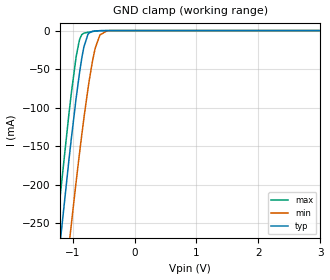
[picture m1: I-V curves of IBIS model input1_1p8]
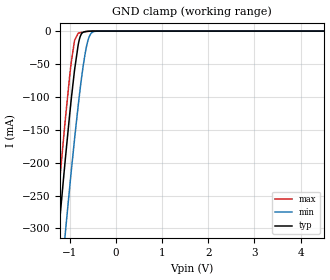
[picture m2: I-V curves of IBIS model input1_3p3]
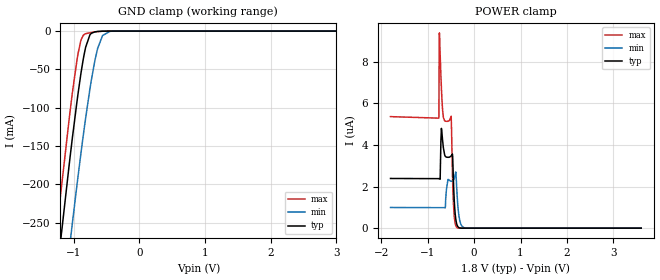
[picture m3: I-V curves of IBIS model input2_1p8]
| Texas Instruments Incorporated
| TLV320ADC5140 Quad-Channel, 768-kHz, Burr-Brown Audio ADC
[IBIS Ver]   4.1
[File name]   tlv320adc5140.ibs
[Date]   05/10/2019
[File Rev]   1.0
[Source]
| Texas Instruments Incorporated.
| Analog-eLab Design Center, HPA
| 12500 TI Blvd
| Dallas, TX -75243
[Notes]   Revision History:
| Rev 1.0: 05/10/2019
| - Initial version of the model
| - Model generated from simulations in SPECTRE
| - C_comp although listed in numerical order of value are
|   obtained from varying PVT conditions. For PVT conditions for
|   each specific value refer the buffer description under
|   respective [Model]. IBIS model user is responsible for using
|   appropriate C_comp to simulate for Signal Integrity.
| - Warnings regarding combined Non-monotonicity of various models have been
|   reviewd and considered minor and can be ignored.
| - Model names with a trailing _1p8 contain the model for 1.8V operation.
|   Model names with a trailing _3p3 contain the model for 3.3V operation.
[Disclaimer]
| This model is designed as an aid for customers of Texas Instruments.
| TI and its licensors and suppliers make no warranties, either expressed
| or implied, with respect to this  model, including the warranties of
| merchantability or fitness for a particular purpose. The model is
| provided solely on an "as is" basis. The entire risk as to its quality
| and performance is with the customer.
| This model is subject to change without notice. Texas Instruments
| Incorporated is not responsible for updating this model.
[Copyright]
(C) Copyright 2019 Texas Instruments Incorporated.All rights reserved.
|  Component TLV320ADC5140RTW 24-Pin WQFN - RTW package
|  Part # TLV320ADC5140RTW
[Component]   TLV320ADC5140RTW
[Manufacturer]  TI
[Package]   |24 WQFN - RTW package
|   typ   min   max
R_pkg   0.05   0.04   0.06
L_pkg   1.0nH   0.8nH   1.2nH
C_pkg   0.2pF   0.16pF   0.24pF
[Pin]  signal_name   model_name   R_pin   L_pin   C_pin
1   AVDD   power   NA   NA   NA
2   AREG   power   NA   NA   NA
3   VREF   nc   NA   NA   NA
4   AVSS   gnd   NA   NA   NA
5   MICBIAS   nc   NA   NA   NA
6   IN1P_GPI1   input1   NA   NA   NA
7   IN1M_GPO1   output   NA   NA   NA
8   IN2P_GPI2   input1   NA   NA   NA
9   IN2M_GPO2   output   NA   NA   NA
10   IN3P_GPI3   input1   NA   NA   NA
11   IN3M_GPO3   output   NA   NA   NA
12   IN4P_GPI4   input1   NA   NA   NA
13   IN4M_GPO4   output   NA   NA   NA
14   SHDNZ   input3   NA   NA   NA
15   ADDR1_MISO   io   NA   NA   NA
16   ADDR0_SCLK   input2   NA   NA   NA
17   SCL_MOSI   od   NA   NA   NA
18   SDA_SSZ   od   NA   NA   NA
19   IOVDD   power   NA   NA   NA
20   GPIO1   io   NA   NA   NA
21   SDOUT   io   NA   NA   NA
22   BCLK   io   NA   NA   NA
23   FSYNC   io   NA   NA   NA
24   DREG   power   NA   NA   NA
|   Model Selectors
[Model Selector] input1
input1_1p8   1.8V   digital Input
input1_3p3   3.3V   digital Input
[Model Selector] input2
input2_1p8   1.8V   digital Input
input2_3p3   3.3V   digital Input
[Model Selector] input3
input3_1p8   1.8V   digital Input
input3_3p3   3.3V   digital Input
[Model Selector] output
output_1p8   1.8V   digital Output
output_3p3   3.3V   digital Output
[Model Selector] io
io_1p8   1.8V   digital I/O
io_3p3   3.3V   digital I/O
[Model Selector] od
od_1p8   1.8V   digital I/O Open-drain
od_3p3   3.3V   digital I/O Open-drain
| Models and submodels in the file (12): input1_1p8 (Input), input1_3p3 (Input), input2_1p8 (Input), input2_3p3 (Input), input3_1p8 (Input), input3_3p3 (Input), output_1p8 (3-state), output_3p3 (3-state), io_1p8 (I/O), io_3p3 (I/O), od_1p8 (I/O_open_drain), od_3p3 (I/O_open_drain)
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|   input1_1p8 Model
[Model]   input1_1p8
Model_type   Input
Vinl = 0.63
Vinh = 1.17
|   typ   min   max
C_comp   0.9411pF   0.9029pF   0.9992pF
[Model spec]
|subparameter
Vinl   0.63   0.567   0.693
Vinh   1.17   1.053   1.287
| Where Nom  PVT is Nominal Process, 1.8V, 27C
|   Fast PVT is Strong Process,  1.98V, -40C
|   Slow PVT is Weak Process,   1.62V, 150C
[Voltage Range]   1.8   1.62   1.98
|Junction Temperature
[Temperature Range]   27   150   -40
[Power Clamp Reference]   1.8   1.62   1.98
[GND Clamp Reference]   0   0   0
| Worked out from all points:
|   GND clamp passes 1 mA (typ) near -0.68 V on its own axis
[GND Clamp]
|   Voltage   I(typ)   I(min)   I(max)
-1.8V     -769.4mA   -875.1mA   -713.6mA
-1.465V   -489.2mA   -598.8mA   -430.8mA
-1.228V   -297mA     -409mA     -236.8mA
-1.206V   -280mA     -392.1mA   -219.8mA
-1.028V   -146mA     -257.5mA   -86.9mA
-892.8mV  -58.07mA   -162.7mA   -13.59mA
-817.2mV  -21.36mA   -114.1mA   -3.368mA
-747mV    -4.455mA   -73.31mA   -2.124mA
-633.6mV  -487.8uA   -22.64mA   -682.1uA
-558mV    -119.9uA   -5.685mA   -166.1uA
-444.6mV  -3.707uA   -331.7uA   -2.899uA
3.6V      0A         0A         0A
[POWER Clamp]
|   Voltage   I(typ)   I(min)   I(max)
-1.8V     0A         0A         0A
0V        0A         0A         0A
3.6V      0A         0A         0A
|   input1_3p3 Model
[Model]   input1_3p3
Model_type   Input
Vinl = 0.8
Vinh = 2
|   typ   min   max
C_comp   0.8273pF   0.7974pF   0.8702pF
| Where Nom  PVT is Nominal Process, 3.3V, 27C
|   Fast PVT is Strong Process,  3.6V, -40C
|   Slow PVT is Weak Process,   3.0V, 150C
[Voltage Range]   3.3   3   3.6
|Junction Temperature
[Temperature Range]   27   150   -40
[Power Clamp Reference]   3.3   3   3.6
[GND Clamp Reference]   0   0   0
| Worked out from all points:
|   GND clamp passes 1 mA (typ) near -0.68 V on its own axis
[GND Clamp]
|   Voltage   I(typ)   I(min)   I(max)
-3.3V     -2.018A    -2.043A    -2.005A
-1.31V    -362.7mA   -474mA     -303.1mA
-1.261V   -323.1mA   -434.8mA   -263.2mA
-1.201V   -276.3mA   -388.4mA   -216mA
-1.092V   -193mA     -305.2mA   -132.8mA
-963.6mV  -101.9mA   -211.4mA   -46.17mA
-894.3mV  -58.92mA   -163.7mA   -14.05mA
-815.1mV  -20.57mA   -112.8mA   -3.303mA
-745.8mV  -4.323mA   -72.66mA   -2.107mA
-636.9mV  -514.1uA   -23.73mA   -714.4uA
-468.6mV  -8.691uA   -624.3uA   -8.339uA
6.6V      0A         0A         0A
[POWER Clamp]
|   Voltage   I(typ)   I(min)   I(max)
-3.3V     0A         0A         0A
0V        0A         0A         0A
6.6V      0A         0A         0A
|   input2_1p8 Model
[Model]   input2_1p8
Model_type   Input
Vinl = 0.63
Vinh = 1.17
|   typ   min   max
C_comp   0.9411pF   0.9029pF   0.9992pF
[Model spec]
|subparameter
Vinl   0.63   0.567   0.693
Vinh   1.17   1.053   1.287
| Where Nom  PVT is Nominal Process, 1.8V, 27C
|   Fast PVT is Strong Process,  1.98V, -40C
|   Slow PVT is Weak Process,   1.62V, 150C
[Voltage Range]   1.8   1.62   1.98
|Junction Temperature
[Temperature Range]   27   150   -40
[Power Clamp Reference]   1.8   1.62   1.98
[GND Clamp Reference]   0   0   0
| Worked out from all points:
|   GND clamp passes 1 mA (typ) near -0.68 V on its own axis
[GND Clamp]
|   Voltage   I(typ)   I(min)   I(max)
-1.8V     -769.4mA   -875.1mA   -713.6mA
-1.465V   -489.2mA   -598.8mA   -430.8mA
-1.228V   -297mA     -409mA     -236.9mA
-1.206V   -280mA     -392.2mA   -219.8mA
-1.028V   -146mA     -257.5mA   -86.91mA
-892.8mV  -58.08mA   -162.7mA   -13.6mA
-817.2mV  -21.37mA   -114.1mA   -3.387mA
-747mV    -4.466mA   -73.31mA   -2.14mA
-633.6mV  -495.5uA   -22.64mA   -692.4uA
-558mV    -124.8uA   -5.691mA   -172.9uA
-444.6mV  -5.169uA   -334.9uA   -5.178uA
3.6V      0A         0A         0A
[POWER Clamp]
|   Voltage   I(typ)   I(min)   I(max)
-1.8V     2.389uA    993.7nA    5.362uA
-757.8mV  2.38uA     986.2nA    5.289uA
-752.4mV  2.379uA    986.2nA    8.477uA
-747mV    2.38uA     986.3nA    9.388uA
-703.8mV  4.797uA    986.3nA    6.738uA
-660.6mV  3.851uA    986.2nA    5.318uA
-493.2mV  3.471uA    2.255uA    5.387uA
-466.2mV  3.56uA     2.268uA    2.627uA
-428.4mV  1.391uA    2.385uA    617.2nA
-369mV    168.3nA    1.712uA    31.42nA
-212.4mV  0A         19.3nA     0A
3.6V      0A         0A         0A
